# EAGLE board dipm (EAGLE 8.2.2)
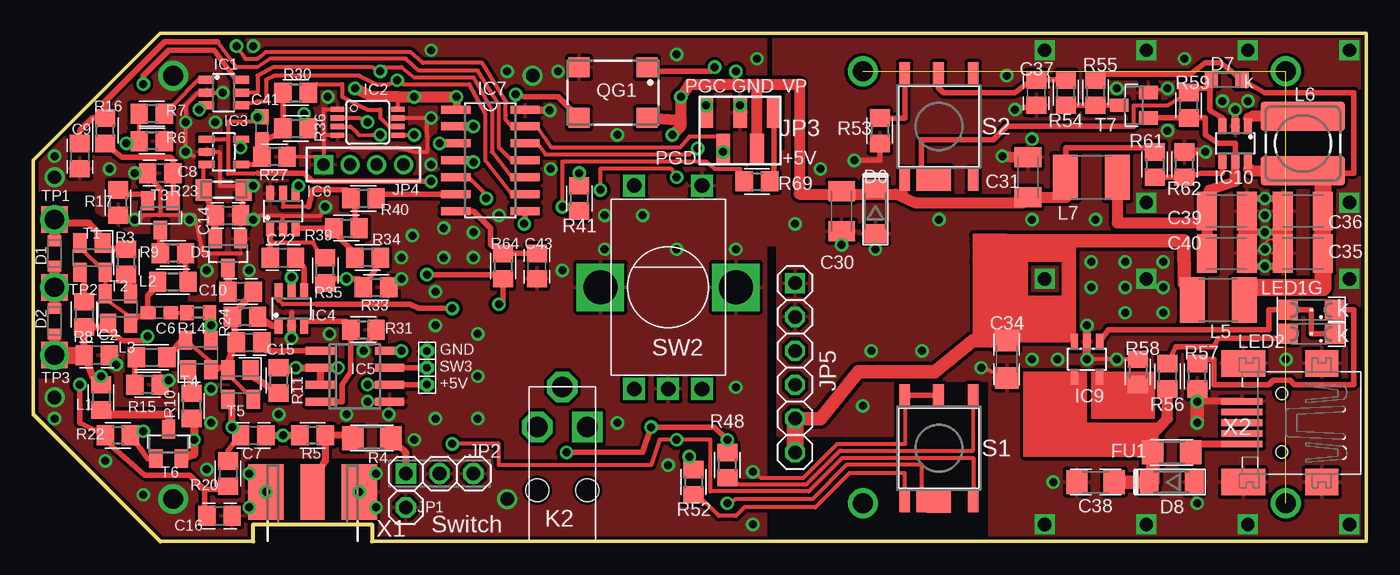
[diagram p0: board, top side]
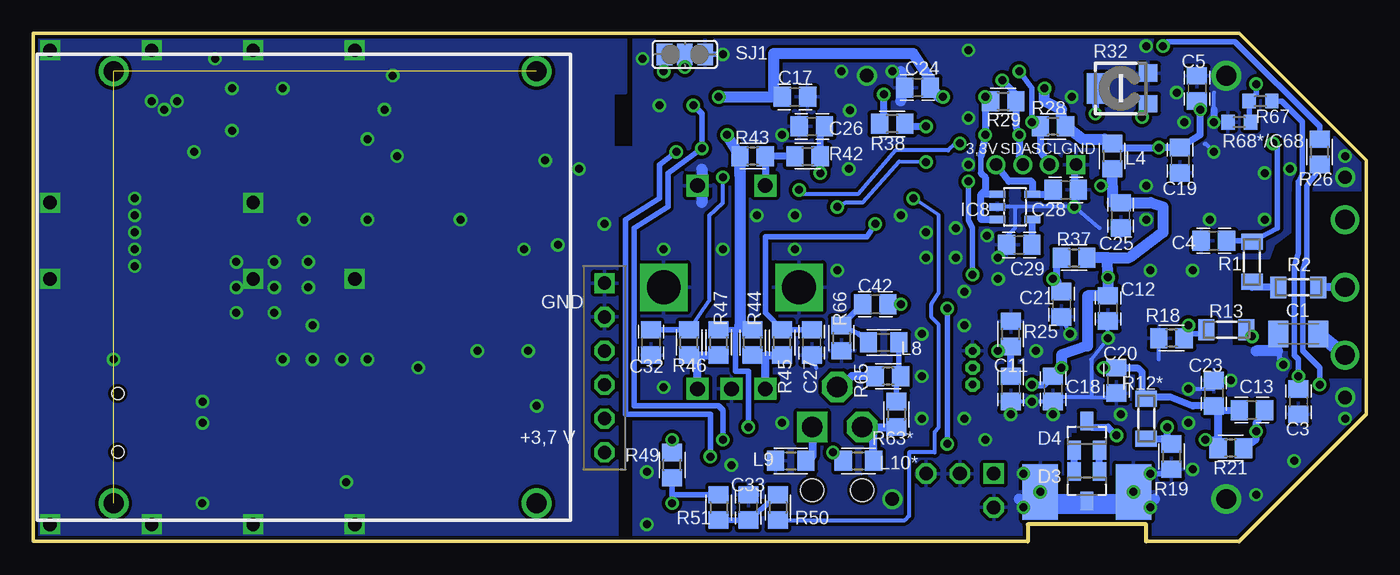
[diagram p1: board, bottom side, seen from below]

Size 100 x 38.1 mm. Coordinates in mm from the lower left corner, seen from the top.
Outline: 0,28.57 9.53,38.09 100,38.09 100,0 25.4,0 25.4,1.27 16.51,1.27 16.51,0 9.53,0 0,9.53 0,28.57
Outline: 0,28.57 9.53,38.1
Copper layers (1*16): Top 0.035mm / dielectric 1.5mm / Bottom 0.035mm
Design rules "default *": minimum track width 6mil, minimum drill 0.35mm, track to track 8mil, track to pad 8mil, pad to pad 8mil, via to via 8mil, smd to smd 0mil, copper to edge 6mil, drill to drill 6mil, minimum pad ring 10mil, minimum via ring 8mil, stop-mask expansion 4mil, vias tented up to drill 0mil, thermal gap 10mil

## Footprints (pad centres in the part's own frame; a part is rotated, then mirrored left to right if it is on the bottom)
C1206K = smd 1.5 x 2: 1 -1.5,0; 2 1.5,0
C0805 = smd 1.3 x 1.5: 1 -0.95,0; 2 0.95,0
C0603 = smd 1.1 x 1: 1 -0.85,0; 2 0.85,0
C1206 = smd 1.6 x 1.8: 1 -1.4,0; 2 1.4,0
C1210K = smd 1.5 x 2.9: 1 -1.5,0; 2 1.5,0
VARICAP = smd 0.8 x 1: A 0.95,0; C -0.95,0
SOT23 = smd 1 x 1.4: 1 -0.95,-1.1; 2 0.95,-1.1; 3 0,1.1
SOD80C = smd 1.4 x 1.8: A 1.7,0; C -1.7,0
DIODE = smd 1 x 1.2: A 1.15,0; C -1.15,0
R1206 = smd 1.6 x 1.803: 1 -1.422,0; 2 1.422,0
SOT23-6 = smd 0.6 x 1.194: 1 -0.95,-1.3; 2 0,-1.3; 3 0.95,-1.3; 4 0.95,1.3; 5 0,1.3; 6 -0.95,1.3
MSOP08 = smd 0.4 x 1: 1 -0.976,-2.263; 2 -0.326,-2.263; 3 0.324,-2.263; 4 0.974,-2.263; 5 0.974,2.262; 6 0.324,2.262; 7 -0.326,2.262; 8 -0.976,2.262
SOT232-5 = smd 0.55 x 1.2: 1 -0.95,-1.3; 2 0,-1.3; 3 0.95,-1.3; 4 0.95,1.3; 5 -0.95,1.3
SO08 = smd 0.6 x 2.2: 1 -1.905,-2.6; 2 -0.635,-2.6; 3 0.635,-2.6; 4 1.905,-2.6; 5 1.905,2.6; 6 0.635,2.6; 7 -0.635,2.6; 8 -1.905,2.6
SO14 = smd 0.6 x 2.2: 1 -3.81,-2.6; 2 -2.54,-2.6; 3 -1.27,-2.6; 4 0,-2.6; 5 1.27,-2.6; 6 2.54,-2.6; 7 3.81,-2.6; 8 3.81,2.6; 9 2.54,2.6; 10 1.27,2.6; 11 0,2.6; 12 -1.27,2.6; 13 -2.54,2.6; 14 -3.81,2.6
1X01 = drill 1.016 octagon: 1 0,0
1X03-S = drill 1.016 square: 1 -2.54,0 | drill 1.016 octagon: 2 0,0; 3 2.54,0
PIN5 = smd 1.016 x 2.2: 1 -1.905,1.33; 2 -0.635,-1.33; 3 0.635,1.33; 4 1.905,-1.33; 5 3.175,1.33
1X04M = drill 0.914 square: 1 -3,0 | drill 0.914: 2 -1,0; 3 1,0; 4 3,0
1X06-S = drill 1 square: 1 -6.35,0 | drill 1 octagon: 2 -3.81,0; 3 -1.27,0; 4 1.27,0; 5 3.81,0; 6 6.35,0
K1501-5 = drill 1.524 square: 1 -1.875,-3.5 | drill 1.524 octagon: 2 0,-6.5; 3 1.875,-3.5 | hole 1.702: -1.875,1.25; 1.875,1.25
0805 = smd 1.3 x 1.5: 1 -0.95,0; 2 0.95,0
COIL1 = smd 1.3 x 1.5: 1 -1.143,0; 2 1.143,0
L1812 = smd 1.9 x 3.4: 1 -1.95,0; 2 1.95,0
POWER-CHOKE_WE-TPC = smd 6.3 x 2.2: 1 0,2.05; 2 0,-2.05
SML1206 = smd 1.5 x 1.5: A 1.75,0; C -1.75,0
SM77H = smd 1.6 x 1.5: 1 -2.55,-1.9; 2 2.55,-1.9; 3 2.55,1.9; 4 -2.55,1.9
MINI_MELF-0204W = smd 1.2 x 1.6: 1 -1.5,0; 2 1.5,0
R0805 = smd 1.3 x 1.5: 1 -0.95,0; 2 0.95,0
R0603 = smd 1 x 1.1: 1 -0.85,0; 2 0.85,0
RTRIMCVR42A = smd 1.3 x 1.4: 1 -1.15,-2.05; 3 1.15,-2.05 | smd 2.3 x 1.5: 2 0,1.8
DTSM-6 = smd 1.676 x 0.813: 1G+ -3.975,2.567; 2G- 3.975,2.567; 3R- -3.975,-2.567; 4R+ 3.975,-2.567; 5 -3.975,1.298; 6 3.975,0.028
SJ_2 = smd 1.168 x 1.6: 1 -1.524,0; 2 0,0; 3 1.524,0
ALPS_EC12E_SW = drill 2.54 square: 1 -5.08,0; 2 5.08,0 | drill 1.1 square: A -2.54,-7.62; B 2.54,-7.62; C 0,-7.62; D -2.54,7.635; E 2.54,7.635
SOT143 = smd 1.2 x 1.44: 1 -0.75,-1.1 | smd 1 x 1.44: 2 0.95,-1.1; 3 0.95,1.1; 4 -0.95,1.1
TP20SQ = smd 2 x 2: TP 0,0
TP18SQ = smd 1.8 x 1.8: TP 0,0
PINHD1X01V = drill 0.559 pad 0.914 octagon: 1 0,0
J502-ND-142-0711-821/826 = smd 4.191 x 1.778: 1 2.115,0 | smd 4.191 x 2.667: G@1 2.115,3.495; G@2 2.115,-3.495 | smd 4.191 x 2.667 bottom: G@3 2.115,3.495; G@4 2.115,-3.495
32005-301 = smd 3.1 x 0.5: 1 3,1.6; 2 3,0.8; 3 3,0; 4 3,-0.8; 5 3,-1.6 | smd 2.5 x 2: M1 -3,-4.45; M2 -3,4.45 | smd 3.3 x 2: M3 2.9,4.45; M4 2.9,-4.45 | hole 0.9: 0,2.2; 0,-2.2

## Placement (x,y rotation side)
C1  100n  [C1206K]  5.08,15.56 0 bottom
C2  10n  [C0805]  4.76,13.97 180 top
C3  4u7  [C0805]  5.08,10.48 90 bottom
C4  100n  [C0805]  11.43,22.54 0 bottom
C5  100n  [C0805]  12.7,33.97 270 bottom
C6  2n2  [C0603]  9.47,17.14 0 top
C7  2n2  [C0805]  16.51,7.94 0 top
C8  470n  [C0805]  9.53,27.62 0 top
C9  47n  [C0805]  3.49,28.89 270 top
C10  2j2  [C0805]  15.56,18.73 0 top
C11  1n  [C0805]  26.67,11.43 90 bottom
C12  4u7  [C0805]  19.37,17.46 270 bottom
C13  100n  [C0805]  8.57,9.84 0 bottom
C14  100  [C0805]  14.61,24.45 0 top
C15  1n  [C0805]  16.19,14.92 0 top
C16  470n  [C0805]  13.97,1.9 180 top
C17  100n  [C0805]  42.86,33.34 0 bottom
C18  100n  [C0805]  23.5,11.43 270 bottom
C19  1u  [C0805]  13.97,28.57 270 bottom
C20  4u7  [C0805]  18.73,12.06 270 bottom
C21  4u7  [C0805]  22.86,17.78 90 bottom
C22  2n2  [C0805]  18.73,21.27 180 top
C23  1u  [C0805]  11.43,11.11 90 bottom
C24  1u  [C0805]  33.66,34.04 0 bottom
C25  1u  [C0805]  18.41,24.45 270 bottom
C26  22n  [C0805]  41.59,31.11 180 bottom
C27  10n  [C0805]  41.59,14.92 270 bottom
C28  4u7  [C0805]  22.54,26.35 180 bottom
C29  10n  [C0805]  26.04,22.23 180 bottom
C30  10u  [C1206K]  60.64,24.77 90 top
C31  10u  [C1206K]  74.61,27.3 270 top
C32  10n  [C0805]  53.66,14.92 270 bottom
C33  10n  [C0805]  46.35,2.54 90 bottom
C34  4u7  [C1206]  73.03,13.65 270 top
C35  10u  [C1210K]  95.25,21.59 180 top
C36  10u  [C1210K]  95.25,24.77 180 top
C37  2u2  [C0805]  75.25,33.66 270 top
C38  4u7  [C1206]  79.69,4.45 180 top
C39  10u  [C1210K]  89.53,24.77 0 top
C40  10u  [C1210K]  89.53,21.59 0 top
C41  2n2  [C0603]  17.14,30.99 90 top
C42  470n  [C0805]  36.83,17.78 180 bottom
C43  4u7  [C0805]  37.78,20.64 90 top
D1  BBY5303  [VARICAP]  1.59,21.59 270 top
D2  BBY5303  [VARICAP]  1.59,16.51 90 top
D3  BAR63-04  [SOT23]  20.95,4.13 180 bottom
D4  BAR63-04  [SOT23]  20.95,7.94 0 bottom
D5  HSMS-2822  [SOT23]  14.61,21.59 180 top
D6  5V1  [SOD80C]  63.18,24.77 270 top
D7  1N4148  [DIODE]  89.53,34.61 180 top
D8  5V6  [SOD80C]  85.41,4.45 0 top
FU1  0,3A  [R1206]  85.41,6.67 180 top
IC1  MCP4726  [SOT23-6]  14.29,33.66 270 top
IC2  MCP4551-103  [MSOP08]  25.08,31.43 270 top
IC3  MCP6271  [SOT232-5]  14.29,29.21 270 top
IC4  NC7SB3157P6  [SOT23-6]  19.37,17.46 0 top
IC5  MC12080D  [SO08]  24.13,12.38 270 top
IC6  TLV3501  [SOT23-6]  18.73,24.77 0 top
IC7  PIC16F1705  [SO14]  34.29,28.57 270 top
IC8  LP2985-3  [SOT232-5]  26.35,25.08 270 bottom
IC9  MCP73831  [SOT232-5]  79.06,13.65 180 top
IC10  MCP1640  [SOT23-6]  90.17,29.85 180 top
JP1  PINHD-1X01_2.54  [1X01]  27.94,2.54 0 top
JP2  [1X03-S]  30.48,5.08 0 top
JP3  [PIN5]  52.39,30.8 0 top
JP4  [1X04M]  24.77,28.26 0 top
JP5  [1X06-S]  57.15,13.02 270 top
K2  [K1501-5]  39.69,5.08 180 top
L1  COIL  [0805]  5.08,10.79 270 top
L2  [COIL1]  10.48,19.47 0 top
L3  [COIL1]  8.89,13.8 0 top
L4  COIL  [0805]  19.05,28.89 90 bottom
L5  1uH  [L1812]  88.9,18.1 180 top
L6  4,7uH  [POWER-CHOKE_WE-TPC]  95.25,29.85 0 top
L7  47uH  [L1812]  79.38,27.3 0 top
L8  [COIL1]  36.2,14.92 0 bottom
L9  [COIL1]  43.18,6.03 0 bottom
L10*  [COIL1]  38.1,6.03 0 bottom
LED1G  HSMF-C115  [SML1206]  95.89,17.36 180 top
LED2  [SML1206]  95.89,15.57 180 top
QG1  SM77H  [SM77H]  43.5,33.66 180 top
R1  33k  [MINI_MELF-0204W]  8.57,20.96 90 bottom
R2  M15  [MINI_MELF-0204W]  5.08,19.05 180 bottom
R3  10  [R0805]  6.99,20.96 90 top
R4  51  [R1206]  25.4,7.75 0 top
R5  47  [R0805]  20.95,7.94 180 top
R6  47k  [R0805]  8.89,30.02 180 top
R7  10k  [R0805]  8.89,32.07 180 top
R8  10  [R0805]  3.81,17.02 270 top
R9  560  [R0805]  10.48,21.59 180 top
R10  10  [R0805]  11.87,10.16 270 top
R11  10  [R0805]  18.41,12.06 270 top
R12*  [MINI_MELF-0204W]  16.51,9.21 270 bottom
R13  22k  [MINI_MELF-0204W]  10.48,15.87 180 bottom
R14  100  [R0603]  12.38,17.14 0 top
R15  560  [R0805]  8.57,11.75 180 top
R16  100k  [R0805]  5.4,30.8 90 top
R17  100  [R0805]  6.35,25.4 270 top
R18  33k  [R0805]  14.61,15.24 180 bottom
R19  33k  [R0805]  14.61,6.35 270 bottom
R20  22k  [R0805]  14.61,5.08 270 top
R21  220k  [R0805]  10.16,6.98 180 bottom
R22  12k  [R0805]  6.35,7.94 180 top
R23  5M6  [MINI_MELF-0204W]  14.29,26.35 180 top
R24  1k  [R0805]  15.88,16.83 180 top
R25  M39  [R0805]  26.67,15.56 90 bottom
R26  220  [R0805]  3.49,29.21 90 bottom
R27  1k  [R0805]  18.1,28.83 180 top
R28  10k  [R0805]  23.5,31.11 180 bottom
R29  10k  [R0805]  27.23,33.02 0 bottom
R30  27k  [R0805]  19.68,33.66 0 top
R31  820  [R0805]  24.77,15.87 0 top
R32  10k  [RTRIMCVR42A]  18.41,33.97 90 bottom
R33  8k2  [R0805]  25.72,19.05 0 top
R34  12k  [R0805]  25.08,21.27 180 top
R35  12k  [R0805]  21.91,20.32 90 top
R36  27k  [R0805]  19.68,30.98 0 top
R37  8k2  [R0805]  21.91,21.27 0 bottom
R38  100  [R0805]  35.56,31.31 180 bottom
R39  1M  [R0805]  23.5,23.5 0 top
R40  100  [R0805]  24.77,25.72 0 top
R41  6k8  [R0805]  40.96,25.72 270 top
R42  2k2  [R0805]  41.91,28.89 0 bottom
R43  5k6  [R0805]  46.04,28.89 180 bottom
R44  10k  [R0805]  46.04,14.92 90 bottom
R45  10k  [R0805]  43.81,14.92 90 bottom
R46  10k  [R0805]  50.8,14.92 90 bottom
R47  10k  [R0805]  48.58,14.92 90 bottom
R48  1k2  [R0805]  52.07,5.71 90 top
R49  10k  [R0805]  52.07,5.71 90 bottom
R50  10k  [R0805]  44.13,2.54 270 bottom
R51  10k  [R0805]  48.58,2.54 270 bottom
R52  680  [R0805]  49.53,4.45 270 top
R53  680  [R0805]  63.5,30.8 270 top
R54  M22  [R0805]  77.47,33.66 90 top
R55  M15  [R0805]  79.69,33.66 270 top
R56  1k2  [R0805]  85.09,12.38 270 top
R57  680  [R0805]  87.31,12.38 90 top
R58  6k8  [R0805]  82.87,12.7 270 top
R59  M82  [R0805]  86.68,32.7 90 top
R61  47k  [R0805]  84.14,28.26 270 top
R62  15k  [R0805]  86.36,28.26 90 top
R63*  220  [R0805]  35.24,9.53 270 bottom
R64  4k7  [R0805]  35.24,20.64 270 top
R65  220  [R0805]  35.88,12.38 180 bottom
R66  220k  [R0805]  39.37,15.24 270 bottom
R67  1k2  [R0603]  7.94,33.02 180 bottom
R68*/C68  220n  [R0603]  9.53,31.43 180 bottom
R69  100  [R0805]  54.29,26.99 0 top
S1  DTSM-6  [DTSM-6]  67.94,6.98 90 top
S2  DTSM-6  [DTSM-6]  67.94,31.11 90 top
SJ1  [SJ_2]  51.12,36.51 180 bottom
SW2  EC12E_SW  [ALPS_EC12E_SW]  47.62,19.05 0 top
T1  BFT182TW  [SOT143]  4.45,21.27 180 top
T2  BFT182TW  [SOT143]  6.35,17.46 0 top
T3  BFR93  [SOT23]  9.53,24.45 180 top
T4  BFT182TW  [SOT143]  12.38,13.97 0 top
T5  BFT182TW  [SOT143]  15.56,11.75 180 top
T6  BSS83P  [SOT23]  10.16,7.3 0 top
T7  2N7002  [SOT23]  82.55,32.7 90 top
TP1  TPSQTP20SQ  [TP20SQ]  1.59,24.13 0 top
TP2  TPSQTP20SQ  [TP20SQ]  1.59,19.05 0 top
TP3  TPSQTP20SQ  [TP20SQ]  1.59,13.97 0 top
TP4  TPTP18SQ  [TP18SQ]  67.94,27.18 0 top
TP5  TPTP18SQ  [TP18SQ]  67.94,3.05 0 top
U$1  PINHD1X1V  [PINHD1X01V]  29.53,11.75 0 top
U$3  PINHD1X1V  [PINHD1X01V]  29.53,14.29 0 top
U$4  PINHD1X1V  [PINHD1X01V]  29.53,13.02 0 top
X1  MCX/SMA  [J502-ND-142-0711-821/826]  20.95,1.59 90 top
X2  MINI-USB  [32005-301]  93.66,8.89 180 top

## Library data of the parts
C1-C43 FU1 L5-L7 R1-R11 R12* R13-R59 R61 R62 R63* R64-R67 R68*/C68 R69 = rcl
D1 D2 D7 IC1-IC4 IC6-IC10 JP3 K2 L1-L4 L8 L9 L10* T3 T6 T7 = pdk1
D3-D6 D8 = diode
IC5 = on-semiconductor; MF: ON SEMICONDUCTOR; MPN: MC12080D; OC_FARNELL: 1607924; OC_NEWARK: 40C2542
JP1 JP2 JP4 JP5 U$1 U$3 U$4 = pinhead-2
LED1G LED2 = led
QG1 = crystal; OC_FARNELL: unknown; OC_NEWARK: unknown
S1 S2 = switch-led
SJ1 = jumper
SW2 = switch-alps_1; MPN: EC12E2424407; OC_FARNELL: 1520813; OC_NEWARK: 74M1068
T1 T2 T4 T5 = transistor
TP1-TP5 = testpad
X1 = con-coax; MF: JOHNSON COMPONENTS; MPN: 142-0711-821; OC_FARNELL: 1019328; OC_NEWARK: 16F3627
X2 = con-cypressindustries; OC_FARNELL: unknown; OC_NEWARK: unknown

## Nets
DAC8: C9.1 IC7.11 R16.2
GND: C1.1 C2.1 C3.1 C4.1 C5.1 C8.1 C9.2 C11.1 C12.2 C14.2 C16.1 C17.2 C18.2 C19.2 C20.2 C21.1 C23.2 C24.1 C25.2 C26.2 C27.2 C28.1 C29.2 C30.1 C31.1 C32.2 C33.2 C34.2 C35.2 C36.2 C37.2 C38.2 C39.2 C40.2 C43.1 D3.3 D5.1 D6.A D8.A IC1.2 IC2.1 IC2.4 IC2.7 IC3.2 IC4.2 IC5.5 IC6.2 IC6.6 IC7.14 IC8.2 IC9.2 IC10.2 JP1.1 JP2.2 JP2.3 JP3.3 JP4.1 JP5.1 JP5.2 L9.1 QG1.2 R6.1 R15.1 R17.2 R18.2 R19.2 R23.1 R25.2 R27.1 R31.2 R32.3 R33.2 R53.2 R57.1 R58.1 R62.2 R66.2 R68*/C68.2 S1.2G- S1.6 SJ1.1 SW2.1 SW2.2 SW2.C SW2.E T7.2 U$3.1 X1.G@1 X1.G@2 X1.G@3 X1.G@4 X2.5 X2.M1 X2.M2 X2.M3 X2.M4
IN+: C41.2 C42.1 IC3.1 R32.1 R64.2
N$1: D1.C R3.2 T1.1 TP1.TP
N$2: C10.1 D5.3
N$3: D1.A D2.A R2.1 TP2.TP
N$4: R8.1 T1.3
N$5: C6.1 L2.1 T1.2 T1.4 T2.2 T2.4
N$6: R3.1 T2.3
N$7: C43.2 IC7.7 R64.1
N$8: IC7.6 R40.2
N$9: L2.2 R9.1
N$10: R1.1 R2.2
N$11: R13.2 R14.2 R18.1 T4.3
N$12: R10.1 T4.1
N$13: C10.2 C15.1 L3.2 R24.2 T4.2 T4.4 T5.2 T5.4
N$14: R17.1 T3.2
N$15: C15.2 IC5.1
N$16: C8.2 R16.1 T3.1
N$17: R9.2 T3.3
N$18: C11.2 IC5.8 R25.1
N$19: IC4.1 R24.1
N$20: IC4.3 IC5.4 R31.1
N$21: C22.2 IC6.1 R35.2
N$22: C22.1 IC4.4
N$23: IC6.3 R34.2 R39.1
N$24: C7.2 D4.3 R5.2
N$25: R4.1 R5.1 X1.1
N$26: IC6.5 R39.2 R40.1
N$27: C21.2 R33.1 R34.1 R35.1 R37.1
N$28: R11.2 T5.1
N$29: L3.1 R15.2
N$30: QG1.1 SJ1.2
N$31: C4.2 R1.2 R6.2 R7.2
N$32: C7.1 R12*.2 R19.1 R20.1 T5.3
N$33: L1.2 T6.3
N$34: C13.2 R21.1 R22.1 T6.1
N$35: IC5.7 U$4.1
N$36: D3.2 D4.1
N$37: D3.1 D4.2
N$38: C6.2 R14.1
N$39: IC1.6 R67.2 R68*/C68.1
N$40: JP2.1 R4.2
N$41: C16.2 R20.2 R22.2 R26.1
N$42: K2.3 L10*.2 R63*.2
N$44: C1.2 C2.2 C3.2 D2.C L1.1 R8.2 R13.1 R67.1 T2.1 TP3.TP
N$49: JP3.5 R69.2
N$57: R49.1 R51.1 S1.5 TP5.TP
N$58: IC1.1 R7.1
N$59: C14.1 D5.2 IC3.3 R23.2
N$60: IC7.4 R41.2 R69.1
N$61: C41.1 IC3.4 R27.2 R30.1 R36.1
N$62: C27.1 IC7.8 R45.2
N$63: IC7.2 R38.1
N$64: C26.1 R41.1 R42.2
N$67: C29.1 IC8.4
N$68: R42.1 R43.1 SW2.D
N$69: QG1.3 R38.2
N$70: R44.1 R45.1 SW2.A
N$71: R46.1 R47.1 SW2.B
N$72: C33.1 R50.1 R51.2
N$73: R32.2 R36.2
N$74: IC10.1 L6.1
N$75: C35.1 C36.1 D7.C IC10.6 L5.1 L6.2 R55.1
N$76: IC2.6 R30.2
N$77: D7.A IC10.3 R59.2 S2.5 TP4.TP
N$78: C39.1 C40.1 IC10.5 L7.2 R59.1 T7.1
N$79: C34.1 IC9.3 JP5.5 JP5.6 L5.2
N$80: K2.2 R65.2
N$81: IC9.5 R58.2
N$82: C37.1 R54.2 S2.6
N$83: IC10.4 R61.2 R62.1
N$84: FU1.1 X2.1
N$85: C38.1 D8.C FU1.2 IC9.4 R56.2
N$86: R54.1 R55.2 T7.3
N$87: IC9.1 LED1G.A LED2.C
N$88: LED1G.C R57.2
N$89: LED2.A R56.1
N$91: R53.1 S2.2G-
N$93: R52.2 S1.1G+
N$94: IC7.13 JP3.2 R26.2 R52.1
N$95: R48.1 S1.4R+
N$96: IC4.6 IC7.12 JP3.1 S1.3R-
N$97: C42.2 L8.1 R66.1
N$100: L8.2 R63*.1 R65.1
N$101: K2.1 L9.2
N$102: C32.1 IC7.3 R46.2
N$103: IC7.5 R50.2
SCL: IC1.5 IC2.2 IC7.10 JP4.2 R28.2
SDA: IC1.4 IC2.3 IC7.9 JP4.3 R29.2
V3.3: C28.2 IC8.5 JP4.4
VCC: C5.2 C17.1 C19.1 C24.2 C30.2 C31.2 D6.C IC1.3 IC2.5 IC2.8 IC3.5 IC7.1 IC8.1 IC8.3 JP3.4 L4.2 L7.1 L10*.1 QG1.4 R28.1 R29.1 R43.2 R44.2 R47.2 R48.2 R49.2 R61.1 S2.1G+ SJ1.3
VDD: C12.1 C13.1 C18.1 C20.1 C23.1 C25.1 IC4.5 IC5.2 IC5.3 IC5.6 IC6.4 L4.1 R10.2 R11.1 R12*.1 R21.2 R37.2 T6.2 U$1.1

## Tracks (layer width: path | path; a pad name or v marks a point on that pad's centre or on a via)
DAC8
  Top 0.305: 13.84,37.46 15.24,35.56 16.83,35.56 17.78,36.2 27.94,36.2 28.89,35.31 33.34,35.31 34.92,32.7 34.92,29.53 35.88,28.57 IC7.11
  Top 0.406: 13.84,37.46 9.84,37.46 5.4,33.02 R16.2 4.44,31.75 3.49,30.8 C9.1
GND  (via drill 0.6, 1, 1.5)
  Top 0.152: 91.03,21.04 C40.2 91.03,21.04 | 91.03,21.04 91.06,21.02 92.69,22.64 93.57,22.64 93.88,22.96 93.88,23.16 | 93.88,23.16 93.88,23.4 | 93.88,23.4 93.78,23.5 | C36.2 93.75,23.53 93.88,23.4 | 93.88,23.4 93.88,23.16 | 91.03,21.04 91.44,20.64 | C35.2 93.75,22.77 93.34,23.18 | C39.2 91.03,25.31 91.44,25.72
  Top 0.305: 10.16,29.85 R6.1 | v14.22,33.66 IC1.2 12.38,33.66 11.43,32.7 v11.43,31.43 v11.43,29.21 12.06,28.89 | v16.51,24.13 15.66,24.13 15.55,24.34 | 18.7,24.42 17.02,24.42 | 18.7,24.42 21.56,24.42 v21.91,25.08 | 18.7,23.62 18.7,24.42 | T7.2 84.14,33.82 v85.09,33.97 | R58.1 81.6,13.65 v79.06,13.65 | R57.1 v87.31,10.49 v87.31,10.48 | C34.2 v71.12,13.02 | C14.2 R23.1 v16.51,26.67 13.97,26.67 13.97,29.21 IC3.2 | 9.51,24.45 12.06,24.45 12.7,21.59 15.56,21.59 | 9.51,26.35 9.51,24.45 | v6.22,13.26 6.03,13.65 | v10.16,12.06 R15.1 | R27.1 21.77,28.89 21.77,30.46 | IC2.4 21.77,30.46 | 9.51,24.45 8.26,24.45 7.94,24.13 | IC2.7 29.52,31.75 29.53,29.21 28.64,29.21 28.18,29.32 27.36,29.53 23.81,29.53 | IC2.1 21.77,32.41 21.77,30.46 | S1.2G- 65.41,10.64 65.41,7.3 60.33,7.3 60.29,7.27 60.28,7.27 57.77,4.76 54.61,4.76 v53.98,5.21
  Top 0.406: v73.66,32.38 C37.2 | R53.2 63.5,28.57 v61.59,28.57 | D6.A v63.18,21.91 | C8.1 9.51,26.35 | v19.37,15.24 IC4.2 19.37,17.14 | R17.2 6.67,24.13 v7.62,24.13 7.94,24.13 | IC5.5 v25.08,10.48 | S1.2G- S1.6 | v24.77,14.29 25.08,14.85 25.19,14.96 25.51,15.35 R31.2
  Top 0.508: IC10.2 v90.17,32.38 | X2.5 v87.31,10.49 | C2.1 v6.22,13.26 | 91.44,20.64 93.34,20.64 | 93.34,23.18 91.44,23.18 | 91.44,25.72 93.34,25.72
  Top 0.61: v87.95,29.21 R62.2 | v79.06,13.65 IC9.2 v79.06,16.19 | IC7.14 v38.73,32.32
  Top 0.813: C30.1 v60.64,22.23 | v72.71,28.89 73.98,28.81 C31.1
  Top 1.016: v87.31,8.89 v87.31,10.49 | v87.31,10.48 R57.1
  Top 1.27: C40.2 C39.2 | 93.66,23.5 93.84,23.18 | C36.2 C35.2
  Bottom 0.305: 15.56,13.65 15.56,14.92 15.55,14.93 | 11.43,32.39 11.43,33.66 | v11.43,29.21 12.06,29.85 12.12,29.79 | 26.35,25.08 26.35,23.5 26.98,22.86 C29.2 | 26.35,25.08 IC8.2 | 20,23.5 v21.91,25.08 | v21.91,25.08 21.91,26.35 C28.1 | JP4.1 21.91,27.94 | v21.91,25.08 26.35,25.08 | C12.2 v19.37,15.24 20.64,13.65 20.64,10.79 | D3.3 20.32,2.54 | C20.2 19.37,10.8 20.64,10.79 | 20.64,10.79 23.18,10.79 C18.2 23.81,10.48 v25.08,10.48 C11.1 | v13.34,11.43 11.43,11.43 C23.2 11.11,12.06 v10.16,12.06 | v22.23,15.56 C21.1 | C27.2 41.27,13.02
  Bottom 0.406: SJ1.1 v48.26,36.51 | v16.19,5.08 14.61,5.08 R19.2 | X1.G@2 24.13,4.02 26.04,3.18 | C1.1 6.48,13.52 v6.22,13.26
  Bottom 0.508: 11.43,32.39 v11.43,31.43 | 21.91,27.94 21.91,26.35
  Bottom 0.813: 26.04,3.18 15.88,3.18 | 6.67,14.29 8.26,14.29 | 34.92,35.24 34.92,33.02 | 49.85,27.94 49.85,25.4
  Bottom 1.016: v16.19,2.54 20.32,2.54 v25.72,2.54
  other vias: 11.75,24.13 1.59,9.21 13.02,5.4 5.4,6.03 10.48,3.18 43.81,8.89 8.26,3.49 13.02,20.32 7.62,27.62 16.19,20.32 23.5,9.53 13.34,8.89 29.84,28.26 10.48,34.92 25.72,5.08 29.84,31.75 18.41,9.53 42.86,21.91 33.34,15.56 54.29,36.2 17.46,3.7 52.7,21.91 48.26,21.91 35.56,35.24 45.72,24.45 42.86,24.45 43.81,30.48 92.39,21.91 86.36,36.2 92.39,24.45 92.39,23.18 87.31,2.86 81.28,13.65 93.98,13.65 76.83,13.65 74.93,30.16 91.12,33.02 89.22,33.02 85.09,30.8 76.52,4.45 66.68,14.29 62.23,10.16 62.87,14.29 79.38,19.05 79.38,20.96 81.92,17.14 84.78,17.14 81.92,19.05 81.92,20.96 84.78,20.96 84.78,19.05 81.28,33.97 5.71,27.94 1.59,28.89 30.16,9.21 30.16,18.73 74.93,13.65 92.39,20.64 92.39,25.71 73.03,34.92 59.05,27.94 57.15,23.81 26.67,9.53 33.34,9.21 33.34,12.38 27.62,21.27 24.45,3.7 28.45,22.92 37.47,34.92 35.56,3.18 53.98,1.27 47.62,5.71 22.1,33.34 27.62,19.69 79.69,24.13 74.93,24.13 67.95,24.13 33.02,23.18 39.69,20.32 28.57,7.62 30.8,23.5 29.84,36.83 16.51,37.15 52.7,11.56 1.59,10.79 1.59,27.3 33.02,21.27 30.8,21.27 34.92,24.45 38.81,27.94 13.65,31.43 30.16,16.19 75.88,1.27 83.5,1.27 75.88,36.83 83.5,36.83 98.74,36.83 98.74,1.27 91.12,1.27 91.12,36.83 98.74,25.4 98.74,19.69 83.5,19.69 83.5,25.4 53.02,32.7 39.37,35.24 75.88,19.69
  pour Top (isolate 0.254): 55.56,38.1 100.01,38.1 100.01,0 71.75,0 71.75,12.06 64.45,12.06 64.45,7.94 55.88,7.94 55.88,22.23 54.93,22.23 54.93,28.26 55.88,28.26 55.88,29.21 56.52,29.21 56.52,33.66 55.56,33.66
  pour Top (isolate 0.254): 9.53,0 16.19,0 16.19,6.35 25.72,6.35 25.72,0 54.93,0 54.93,38.1 9.53,38.1 0,28.57 0,26.35 4.76,26.35 4.76,24.77 7.3,23.18 9.53,23.18 9.53,22.23 11.75,22.23 11.75,18.1 14.29,18.1 14.29,13.97 4.45,13.97 4.45,12.06 0,12.06 0,9.53
  pour Top: 78.74,16.51 85.41,16.51 85.41,21.59 78.74,21.59
  pour Bottom (isolate 0.254): 56.2,0 100.01,0 100.01,38.1 55.56,38.1 55.56,33.66 56.52,33.66 56.52,29.53 54.93,29.53 54.93,24.45 56.2,24.45
  pour Bottom (isolate 0.254): 25.4,0 54.93,0 54.93,38.1 9.53,38.1 0,28.57 0,26.35 5.71,26.35 5.71,23.18 6.99,22.23 7.3,21.27 10.16,21.27 10.16,14.6 4.45,14.6 4.45,12.06 0,12.06 0,9.53 9.53,0 16.51,0 16.51,1.9 18.41,1.9 18.41,5.08 20.64,5.08 20.64,8.25 22.23,8.25 22.23,5.08 23.5,5.08 23.5,1.9 25.4,1.9
IN+  (via drill 0.6)
  Top 0.305: IC3.1 14.29,30.16 14.61,30.16 | 14.61,30.16 14.61,27.56 16.51,27.56 16.83,27.62 | 14.61,30.16 14.61,31.5 16.51,31.5 v16.83,31.81 16.98,31.81 C41.2
  Top 0.406: v29.84,26.99 20.95,26.99 20.32,27.62 16.83,27.62 | v29.53,20 34.93,20.01 R64.2 35.24,18.1 v34.92,17.78
  Bottom 0.305: R32.1 16.19,32.7 16.51,32.5
  Bottom 0.406: v29.53,20 29.53,23.5 29.84,24.13 v29.84,26.99 | C42.1 v34.92,17.78
  Bottom 0.508: 16.51,32.5 v16.83,31.81
N$1  (via drill 1.45)
  Top 0.305: 1.58,23.81 TP1.TP
  Top 0.508: TP1.TP 1.8,24.13 1.85,23.87 4.17,23.87 4.88,23.16 T1.1 5.66,21.91 R3.2
  Top 0.813: D1.C 1.59,23.81 1.58,23.81
  other vias: 1.59,24.13
N$2
  Top 0.508: D5.3 C10.1
N$3  (via drill 1.45)
  Top 0.305: 1.27,19.05 TP2.TP | TP2.TP 1.59,18.1 | 1.59,19.69 TP2.TP
  Top 0.813: D2.A TP2.TP | TP2.TP D1.A
  Bottom 0.61: TP2.TP R2.1
  other vias: 1.59,19.05
N$4
  Top 0.305: 3.81,19.86 T1.3
  Top 0.406: R8.1 3.81,19.86
N$5
  Top 0.305: T1.2 3.5,22.07 T1.4 5.39,20.15 T2.4 5.55,18.1 7.3,16.83 7.3,16.68 T2.2 | 7.3,16.83 T2.2 | 8.99,17.35 C6.1 8.57,17.14 | T2.2 7.52,16.68 | 9.53,19.37 L2.1
  Top 0.406: 7.52,16.68 C6.1 | 8.57,17.14 8.57,18.42 9.53,19.37
N$6
  Top 0.305: T2.3 7.3,19.79 7.2,19.79 R3.1
N$7
  Top 0.406: C43.2 R64.1 34.29,22.23 34.29,23.5 33.02,24.77 IC7.7
N$8
  Top 0.305: R40.2 26.35,26.04
  Top 0.406: 26.35,26.04 IC7.6
N$9
  Top 0.406: R9.1 11.43,20 L2.2
N$10
  Bottom 0.305: 8.57,19.05 R1.1
  Bottom 0.508: R2.2 8.57,19.05
N$11  (via drill 0.6)
  Top 0.305: R14.2 13.33,17.36 | v13.34,16.19 v13.33,16.19
  Top 0.406: 13.33,17.36 v13.33,16.19 T4.3
  Bottom 0.305: R13.2 11.74,15.56 | 13.02,15.56 13.34,15.24 R18.1 13.34,15.56 v13.34,16.19
  Bottom 0.406: 11.74,15.56 13.02,15.56
N$12
  Top 0.305: T4.1 11.5,12.55
  Top 0.508: 11.5,12.55 11.75,12.06 11.75,11.11 R10.1
N$13
  Top 0.305: 13.33,13.02 T4.2 | T4.2 13.33,12.85 | C15.1 15.09,14.78 | C15.1 15.24,14.6 | C15.1 | T4.2 14.52,12.91 13.57,13.25 T4.4 | 11.19,15.56 11.59,15 11.75,14.92 11.75,15.39 T4.4 | 14.59,13.19 T5.2 14.61,12.55 T5.4 | 11.43,15.39 T4.4
  Top 0.508: 14.52,12.91 15.09,14.78 | C15.1 R24.2 C10.2 | T4.2 14.59,13.19 | L3.2 11.43,15.39
N$14
  Top 0.305: R17.1 6.99,26.03 | 8.57,26.04 8.72,25.4 T3.2
  Top 0.406: 6.99,26.03 8.57,26.04
N$15
  Top 0.305: 17.46,14.29 C15.2
  Top 0.406: IC5.1 17.46,14.29
N$16
  Top 0.305: R16.1 5.73,29.53
  Top 0.406: 10.48,26.03 C8.2 10.47,28.58 10.25,28.8 6.68,28.8 5.73,29.53
  Top 0.508: T3.1 10.48,26.03
N$17
  Top 0.508: T3.3 9.53,22.55 R9.2
N$18  (via drill 0.6)
  Top 0.305: IC5.8 v27.62,14.29
  Bottom 0.305: R25.1 v27.62,14.29
  Bottom 0.508: C11.2 R25.1
N$19
  Top 0.508: R24.1 17.9,16.19 IC4.1
N$20
  Top 0.305: 23.81,16.19 R31.1 23.69,16.19 | 23.69,16.19 R31.1 | IC4.3 20.5,16.31 20.6,16.51 | 23.47,16.51 23.69,16.19
  Top 0.406: IC5.4 23.18,10.48 23.18,11.75 23.81,12.7 23.81,16.19 | 20.6,16.51 23.47,16.51
N$21
  Top 0.305: R35.2 21.27,21.91 21.01,22.43 17.78,22.43 17.78,22.54 | 17.78,21.59 C22.2
  Top 0.406: 17.78,21.59 17.78,22.54 | 17.78,22.43 IC6.1
N$22
  Top 0.305: C22.1
  Top 0.406: IC4.4 20.32,20.52 C22.1
N$23
  Top 0.305: R39.1 22.86,22.86 | 24.13,21.59 R34.2
  Top 0.406: 22.86,22.86 24.13,21.59 | R39.1 20.32,23.5 IC6.3
N$24  (via drill 0.6)
  Top 0.508: C7.2 v18.73,7.94 R5.2
  Bottom 0.508: D4.3 20.95,8.89 20.64,8.57 19.37,8.57 v18.73,7.94
N$25
  Top 0.305: X1.1 20.96,4.79 20.95,4.47 | R5.1
  Top 0.508: R4.1 23.5,7.94 R5.1 | R5.1 21.91,6.03 20.95,4.47
N$26
  Top 0.305: IC6.5 18.73,25.08 20.64,25.08 | R40.1 23.5,26.35
  Top 0.406: 23.5,26.35 20.95,26.35 20.64,25.08 | R39.2 24.13,24.13 24.13,25.08 R40.1
N$27  (via drill 0.6)
  Top 0.305: 25.98,20.9 26.3,20.9 26.35,20.95 R34.1
  Top 0.406: R35.1 22.23,19.69 v23.5,19.69 24.45,19.69 R33.1 25.98,20.9
  Bottom 0.305: R37.1 23.23,21.27
  Bottom 0.508: 23.23,19.7 v23.5,19.69 | 23.23,19.7 C21.2 | 23.23,21.27 23.23,19.7
N$28
  Top 0.305: R11.2 18.41,10.8 | T5.1 16.68,12.21
  Top 0.508: 16.68,12.21 R11.2
N$29
  Top 0.305: L3.1 7.62,13.65
  Top 0.406: 7.62,13.65 R15.2
N$30  (via drill 0.6)
  Top 0.305: 46.67,35.24 QG1.1
  Top 0.406: v51.12,35.56 50.8,35.24 46.67,35.24
  Bottom 0.406: SJ1.2 v51.12,35.56
N$31  (via drill 0.6)
  Top 0.305: v6.99,29.85 7.94,30.16 | 7.94,30.16 R7.2 | 8.26,30.16 7.94,30.16
  Top 0.406: R6.2 v6.99,29.85
  Bottom 0.406: v6.99,29.85 6.67,29.53 6.67,23.5 R1.2 8.66,22.54 C4.2
N$32  (via drill 0.6)
  Top 0.305: T5.3 14.61,10.48 | 15.24,8.25 C7.1 15.49,8.01
  Top 0.406: R20.1 14.61,6.81 15.49,8.01
  Top 0.508: 14.61,10.48 14.92,9.84 v14.92,8.57 15.24,8.25
  Bottom 0.508: 14.92,7.71 v14.92,8.57 | R12*.2 14.92,7.71 | 14.92,7.71 R19.1
N$33
  Top 0.508: 5.4,9.84 L1.2
  Top 0.61: L1.2 5.4,9.53 10.16,9.53 T6.3
N$34  (via drill 0.6)
  Top 0.305: R22.1 6.99,8.25 6.98,8.26 7.62,8.26 v8.26,8.25
  Top 0.406: T6.1 8.57,6.2 R22.1
  Bottom 0.508: C13.2 8.26,8.89 v8.26,8.25 8.26,7.62 R21.1
N$35
  Top 0.406: IC5.7 U$4.1
N$36
  Bottom 0.508: D3.2 D4.1
N$37
  Bottom 0.508: D3.1 D4.2
N$38
  Top 0.305: C6.2 R14.1
N$39  (via drill 0.6)
  Top 0.406: IC1.6 15.24,34.6 15.25,34.6 15.12,34.74 13.56,36.83 10.16,36.83 8.26,34.92 v8.26,34.29
  Bottom 0.406: R68*/C68.1 8.79,31.54 R67.2 8.26,33.55 v8.26,34.29
N$40
  Top 0.508: R4.2 27.94,6.67 JP2.1
N$41  (via drill 0.6)
  Top 0.305: 5.34,7.99 5.02,8 R22.2 | 14.61,3.9 R20.2
  Top 0.406: R22.2 3.49,8.89 v3.49,11.75 | 5.34,7.99 5.87,7.15 8.36,4.97 11.72,4.97 12.8,3.9 12.85,3.9 | 12.85,3.9 14.61,3.9 | C16.2 12.85,2.37 12.85,3.9
  Bottom 0.406: v3.49,11.75 3.49,13.02 4.76,14.29 4.76,20.32 4.45,21.27 4.45,26.67 3.49,27.94 R26.1
N$42
  Bottom 0.406: 36.96,8.56 37.13,8.57
  Bottom 0.61: R63*.2 37.13,8.57 37.19,8.57 K2.3 | L10*.2 36.96,8.56
N$44  (via drill 0.6, 1.45)
  Top 0.305: 1.9,14.6 TP3.TP | v5.08,12.38 5.39,11.75 L1.1 | 5.4,16.25 T2.1
  Top 0.406: 5.31,16.07 6.72,15.06 8.26,15.06 v8.57,15.37
  Top 0.508: v5.08,12.38 4.45,12.38 C2.2 3.81,15.75 R8.2 5.31,16.07 T2.1
  Top 0.813: TP3.TP D2.C
  Top 1.27: TP3.TP C2.2
  Bottom 0.305: R13.1 v8.57,15.37
  Bottom 0.406: v5.08,12.38 5.08,13.65 5.4,13.97 5.4,20.64 5.08,21.59 5.08,26.97 4.8,27.56 4.8,31.47 6.35,33.02 R67.1
  Bottom 0.508: C3.2 v5.08,12.38
  Bottom 1.016: C1.2 TP3.TP
  other vias: 1.59,13.97
N$45  (via drill 1.5)  (2 unrouted)
  other vias: 62.23,35.24 93.98,35.24 93.98,2.86
N$46  (via drill 1.5)
  other vias: 62.23,2.86
N$49
  Top 0.406: JP3.5 55.56,26.67 R69.2
N$57  (via drill 0.6)
  Top 0.305: v52.07,2.86 52.7,3.18 58.45,3.18 61.01,5.74 66.65,5.74 S1.5 67.91,3.01 TP5.TP
  Bottom 0.406: 52.07,3.49 R49.1 | 52.07,3.49 v52.07,2.86 | 52.07,3.49 51.12,3.49 50.8,3.49 R51.1
N$58
  Top 0.305: IC1.1 12.38,34.6 10.48,32.7 R7.1
N$59
  Top 0.305: D5.2 13.65,23.01 | 13.65,24.13 C14.1 | R23.2 12.79,28.14 IC3.3
  Top 0.508: 13.65,23.01 13.65,24.13 | C14.1 R23.2
N$60  (via drill 0.6)
  Top 0.305: 31.49,28.57 IC7.4 | R41.2 v39.69,25.08 39.69,28.5 50.48,28.5 51.12,27.94 53.02,27.94 53.02,26.67 R69.1
  Top 0.406: IC7.4 v33.02,28.45
  Bottom 0.305: v33.02,28.45 35.04,28.47 37.78,25.4 39.05,25.4 v39.69,25.08
N$61
  Top 0.305: 17.18,28.29 R27.2 17.46,29.21 | R36.1 18.59,30.66 | C41.1 17.25,29.95 17.46,30.16
  Top 0.406: IC3.4 17.18,28.29 | R30.1 18.73,31.43 R36.1 | 18.59,30.66 17.46,30.16 17.46,29.21
N$62  (via drill 0.6)
  Top 0.305: 36.89,24.67 IC7.8 | 36.89,23.87 v36.83,23.81
  Top 0.406: IC7.8 36.89,23.87
  Bottom 0.406: C27.1 R45.2 45.09,17.14 45.09,22.86 37.47,22.86 v36.83,23.81
N$63  (via drill 0.6)
  Top 0.305: IC7.2 31.75,31.11
  Top 0.406: IC7.2 v33.02,31.11
  Bottom 0.508: R38.1 34.29,31.11 v33.02,31.11
N$64  (via drill 0.6)
  Top 0.305: R41.1 v40.96,27.62
  Bottom 0.305: R42.2
  Bottom 0.508: R42.2 40.96,30.8 C26.1 | v40.96,27.62 R42.2
N$67
  Bottom 0.508: C29.1 25.05,23.53 IC8.4
N$68
  Bottom 0.305: SW2.D
  Bottom 0.508: R42.1 R43.1 SW2.D
N$69  (via drill 0.6)
  Top 0.406: QG1.3 39.36,33.35 36.83,33.34 v36.2,33.53
  Bottom 0.508: R38.2 36.32,31.31 36.2,31.43 v36.2,33.53
N$70
  Bottom 0.406: 45.02,13.97 R44.1
  Bottom 0.61: SW2.A 45.09,13.65 45.02,13.97 R45.1
N$71
  Bottom 0.305: R47.1 48.9,13.95 | R46.1 51.12,13.95
  Bottom 0.61: SW2.B 50.16,13.97 | 50.16,13.97 R46.1 | 50.16,13.97 R47.1
N$72
  Bottom 0.406: R51.2 C33.1 R50.1
N$73  (via drill 0.6)
  Top 0.305: R36.2 20.32,30.97 v20.32,32.07
  Bottom 0.305: R32.2 20.32,33.66
  Bottom 0.508: 20.32,33.66 v20.32,32.07
N$74
  Top 0.406: IC10.1 91.12,31.75 91.19,31.75
  Top 0.813: L6.1 91.5,31.89 91.19,31.75
N$75
  Top 0.305: 97.75,27.62 96.75,27.89 | 79.96,35.04 R55.1
  Top 0.406: 97.75,27.62 99.06,27.62 99.06,33.66 92.39,33.66 D7.C 89.1,35.88 87.95,35.88 86.82,35.04 79.96,35.04 | IC10.6 91.12,27.8 91.5,27.8
  Top 0.813: L6.2 91.5,27.8 91.19,27.94
  Top 1.016: L5.1 90.85,19.05 90.81,19.05
  Top 1.27: 90.81,19.05 96.75,19.05 C35.1 C36.1 96.75,27.89 L6.2 95.25,27.64
N$76
  Top 0.305: R30.2 21.27,34.29 23.18,34.29 23.18,33.34 25.08,32.38 26.04,32.38 26.04,31.75 26.67,31.11 IC2.6
N$77
  Top 0.305: 82.55,31.11 82.55,32.7 85.11,32.7 R59.2 | R59.2 | R59.2 | TP4.TP 66.69,27.18 S2.5
  Top 0.406: 82.55,31.11 73.03,31.11 72.05,30.14 66.65,30.14 S2.5 | R59.2 86.68,33.97 88.27,33.97 D7.A 88.27,33.66 88.27,32.38 88.39,32.27 89.22,31.75 IC10.3
N$78
  Top 0.305: R59.1 86.74,31.37 86.36,31.75
  Top 0.406: IC10.5 90.17,29.85 88.9,29.85 87.95,30.48 87.95,31.75 R59.1 | T7.1 86.36,31.75
  Top 0.508: 90.17,27.62 IC10.5
  Top 0.813: 90.17,27.62 90.17,26.99 88.27,26.35 88.03,25.8 C39.1 88.03,23.88 | 88.03,23.88 C40.1 | L7.2 81.33,23.88 88.03,23.88
N$79
  Top 0.254: 78.11,22.54 | 78.11,14.6 78.11,14.89 78.11,22.69 78.11,22.86
  Top 0.305: L5.2 86.68,18.1 86.68,19.37 | IC9.3 78.11,14.89 | 78.11,22.54 78.11,22.69
  Top 1.016: JP5.5 59.05,9.21 61.91,12.7 67.63,12.7 70.48,15.05 C34.1 73.03,22.54 78.11,22.54 86.31,22.54 86.36,19.37 86.36,19.69 L5.2
  Top 1.27: JP5.5 JP5.6
N$80
  Bottom 0.61: R65.2 38.59,12.38 K2.2
N$81
  Top 0.305: R58.2 80.01,11.75 IC9.5
N$82
  Top 0.305: 74.93,34.63 C37.1
  Top 0.406: C37.1 R54.2 | S2.6 67.92,34 68.26,33.66 73.63,33.66 74.93,34.63
N$83
  Top 0.305: 89.22,28.59 IC10.4 89.2,28.57
  Top 0.406: R61.2 R62.1 87.63,27.62 89.22,27.62 89.2,28.57
N$84
  Top 0.305: 87.32,7.29 FU1.1
  Top 0.508: X2.1 87.32,7.29
N$85
  Top 0.305: IC9.4 78.11,8.22 83.82,8.25 83.82,8.02 83.91,7.93
  Top 0.813: 83.91,7.93 85.09,9.21 R56.2
  Top 1.016: C38.1 D8.C 83.99,4.45 FU1.2 83.91,6.67 83.91,7.93
N$86
  Top 0.305: T7.3
  Top 0.406: R54.1 R55.2 T7.3
N$87
  Top 0.406: IC9.1 80.64,15.87 92.71,15.87 92.71,17.36 LED1G.A 95.89,17.36 95.89,15.57 LED2.C
N$88
  Top 0.305: 87.31,13.65 R57.2
  Top 0.406: LED1G.C 99.06,17.36 99.06,11.75 94.61,11.75 94.3,12.09 93.03,12.09 92.71,11.75 88.58,11.75 88.58,13.65 87.31,13.65
N$89
  Top 0.406: R56.1 85.72,14.6 88.58,14.6 88.9,15.24 94.14,15.24 LED2.A
N$91
  Top 0.406: R53.1 65.38,31.75 S2.2G-
N$93
  Top 0.305: S1.1G+ 65.38,5.14 61.28,5.14 58.67,2.54 53.34,2.54 52.7,1.9 51.44,1.9 49.85,3.49 R52.2
N$94  (via drill 0.6)
  Top 0.305: v15.24,37.15 15.88,36.2 16.83,36.2 17.46,36.7 28.26,36.7 29.21,35.88 33.66,35.88 35.43,33.02 35.43,31.63 | v51.75,29.21 51.75,30.35 49.21,30.35 48.51,29.53 38.89,29.53 37.78,31.11 37.09,31.11 | 35.43,31.63 35.43,31.94 | IC7.13 35.88,31.11 35.43,31.63
  Top 0.406: v49.21,6.35 R52.1 | 37.09,31.11 IC7.13 | JP3.2 51.81,29.47 v51.75,29.21
  Bottom 0.406: v15.24,37.15 14.92,37.46 9.84,37.46 3.49,31.11 R26.2 | v49.21,6.35 49.21,9.53 55.56,9.53 55.56,24.13 53.02,25.72 53.02,28.26 v51.75,29.21
N$95
  Top 0.305: S1.4R+ 70.51,6.79 60.53,6.79 60.5,6.76 60.49,6.76 57.98,4.25 53.02,4.25 R48.1
N$96  (via drill 0.6)
  Top 0.305: S1.3R- 70.51,6.25 60.7,6.25 58.19,3.75 50.8,3.75 50.8,7.62 v48.26,7.62 46.99,7.62 46.35,5.71 34.92,5.71 34.92,7.3 v31.43,7.3 | IC4.6 18.41,18.61 | 21.27,17.78 18.73,17.78 18.42,18.1 | 37.78,29.85 38.42,29.02 49.21,29.02 v49.85,29.46
  Top 0.406: 18.42,18.1 IC4.6 | 21.27,17.78 28.26,17.78 28.89,17.46 v31.43,17.46 | IC7.12 37.78,29.85 | v50.48,32.7 50.42,32.07 JP3.1
  Bottom 0.406: v31.43,7.3 v31.43,17.46 | v48.26,7.62 48.26,9.84 48.58,10.16 54.93,10.16 54.93,23.5 52.39,25.08 52.39,27.62 v49.85,29.46 49.85,32.07 v50.48,32.7
N$97
  Bottom 0.406: L8.1 38.1,15.56 R66.1 C42.2
N$100
  Bottom 0.406: L8.2 35.05,13.02 R65.1 35.24,12.38 R63*.1
N$101
  Bottom 0.406: 41.56,6.35 L9.2
  Bottom 0.61: K2.1 41.56,6.35
N$102  (via drill 0.6)
  Top 0.305: v48.26,27.3 47.87,27.94 42.52,27.94 42.52,26.33 v42.55,26.35 | IC7.3 v30.48,29.85
  Bottom 0.305: v48.26,27.3 48.26,25.38 49.3,24.43 49.3,18.08 R46.2 | v30.48,29.85 30.82,29.85 31.38,29.32 35.32,29.32 38.14,26.04 42.23,26.04 v42.55,26.35
  Bottom 0.406: R46.2 C32.1
N$103  (via drill 0.6)
  Top 0.305: v33.97,25.72 33.78,25.91 33.78,26.17 32.64,27.3 IC7.5
  Bottom 0.305: R50.2 34.61,1.59 34.29,1.9 34.29,6.67 32.38,6.67 32.38,8.2 32.11,8.52 32.11,16.29 32.61,16.79 32.61,17.82 32.07,18.68 32.07,24.45 v33.97,25.72
SCL  (via drill 0.6)
  Top 0.305: IC1.5 16.83,33.66 16.83,34.92 18.01,35.56 25.4,35.56 v26.04,35.24 26.35,35.56 27.62,35.56 28.57,34.8 33.02,34.8 34.42,32.38 34.42,29.21 35.88,27.3 IC7.10 | IC2.2 24.45,31.75 v25.07,31.44
  Bottom 0.305: 24.45,31.12 v25.07,31.44 24.44,31.43 R28.2
  Bottom 0.406: v25.07,31.44 25.08,32.07 25.08,33.97 v26.04,35.24
  Bottom 0.508: JP4.2 24.45,29.26 24.45,31.12
SDA  (via drill 0.6)
  Top 0.305: IC1.4 16.83,33.02 17.46,33.02 17.46,34.61 18.1,34.92 24.45,34.92 25.72,34.29 26.69,34.29 v27.3,34.58 27.3,34.61 27.76,34.29 32.7,34.29 33.91,32.07 33.91,28.57 35.88,26.04 IC7.9 | IC2.3 23.81,31.11 24.13,30.8 24.44,30.47 25.4,30.48 v26.04,30.48
  Bottom 0.406: v27.3,34.58 26.36,33.63 R29.2
  Bottom 0.508: R29.2 26.28,31.11 v26.04,30.48 26.04,28.85 JP4.3
V3.3
  Bottom 0.305: 25.05,26.96 25.08,26.99 | 23.81,26.03 C28.2
  Bottom 0.508: 25.05,26.96 IC8.5 23.81,26.03 | 25.08,26.99 26.81,26.99 JP4.4
VCC  (via drill 0.6)
  Top 0.254: C30.2 60.01,26.04
  Top 0.305: IC3.5 15.55,30.16 v15.56,29.53 | IC2.8 27.39,33.36 27.39,33.34 | IC2.5 27.94,30.46 v28.57,30.48 | IC7.1 31.46,32.38 31.75,32.41 | IC1.3 12.99,32.67 v12.45,32.38 | D6.C 63.13,26.46 64.72,26.04
  Top 0.406: 77.47,27.94 77.47,29.53 83.5,29.53 R61.1 | 65.38,27.1 S2.1G+ 65.38,25.72 66.12,25.4 | R48.2 v52.07,7.62 51.12,8.57 v46.35,8.57 45.72,6.67 v40.01,6.67 | 52.7,34.29 v52.7,35.24
  Top 0.61: v31.75,33.34 31.75,32.41
  Top 0.813: v24.13,33.97 25.4,33.34 27.39,33.34 v28.57,33.34 v31.75,33.34 | 54.29,34.29 52.7,34.29 49.21,34.29 v48.58,33.34 48.58,31.91 | L7.1 77.47,27.94 77.47,25.8 C31.2 74.3,25.4 66.12,25.4 64.72,26.04 60.01,26.04 57.47,26.04 57.47,34.29 54.29,34.29 | JP3.4 54.29,34.29 | 48.58,31.91 48.58,31.11 v47.94,30.48 | QG1.4 48.29,31.62 48.58,31.91
  Bottom 0.305: 19.62,30.16 L4.2 | 44.45,33.34 C17.1 | IC8.1 | R29.1 v28.57,33.34 | R44.2 46.35,15.56 46.99,16.19 47.31,15.87 | R48.2 v52.07,7.62
  Bottom 0.406: 28.89,28.89 28.89,27.62 | R47.2 47.31,15.87 | 47.31,15.87 R44.2 | L10*.1 39.05,6.35 v40.01,6.67 | 47.31,15.87 47.31,12.76 46.35,12.76 v46.35,8.57 | SJ1.3 52.64,35.31 v52.7,35.24
  Bottom 0.508: L4.2 18.73,29.53 v15.56,29.53 C19.1 12.45,30.48 v12.45,32.38 C5.2 | IC8.3 28.89,24.13 28.89,26.04 | IC8.1 28.89,26.04 | v28.57,33.34 v28.57,30.48 28.89,28.89 | 28.89,27.62 28.57,27.3 28.57,26.35 28.89,26.04
  Bottom 0.813: 44.45,33.34 44.45,36.58 33.97,36.58 32.7,34.67 C24.2 32.01,33.34 v31.75,33.34 | 46.99,27.46 46.99,16.19 | R43.2 | R43.2 46.99,27.46 | v24.13,33.97 24.13,33.02 22.86,32.38 22.86,31.75 R28.1 21.27,30.16 19.62,30.16 | v48.58,33.34 C17.1 | v47.94,30.48 R43.2 | R43.2 46.99,27.46
VDD  (via drill 0.6)
  Top 0.305: R11.1 18.73,12.7 | IC6.4 19.68,26.23 v19.89,26.67
  Top 0.406: IC5.6 U$1.1
  Top 0.508: IC5.2 v19.68,13.02 18.73,12.7 | R10.2 12.06,9.21 | IC4.5 v19.37,19.8 | IC5.2 IC5.3 | IC5.2 v22.86,13.02 | v25.08,11.75 IC5.6
  Top 0.61: 12.06,9.21 v12.06,7.62 12.06,6.52 T6.2
  Bottom 0.305: R12*.1 16.82,11.11 | 16.51,10.48 R12*.1 | 16.51,11.11 R12*.1 | 11.15,9.84 11.43,9.84 | 19.05,25.4 C25.1 | 19.05,26.67 19.05,26.68
  Bottom 0.406: 11.11,7.62 11.11,7.61
  Bottom 0.508: v19.68,13.02 C20.1 17.14,13.01 16.83,12.7 16.82,11.11 | 16.19,10.92 16.51,10.48 | 11.43,9.84 C23.1 12.93,10.16 12.94,10.17 13.03,10.17 14.61,10.79 16.42,10.79 R12*.1 | 11.15,9.84 C13.1 | v25.08,11.75 24.13,11.74 C18.1 | v19.89,26.67 19.05,26.67 | v12.06,7.62 11.11,7.62
  Bottom 0.61: R21.2 11.11,7.61 11.11,10.16 C23.1
  Bottom 0.813: L4.1 19.05,26.68 19.05,25.4 | C25.1 16.18,25.4 15.24,25.08 15.24,23.18 17.78,21.27 19.4,21.27 | 19.4,21.27 R37.2 | 19.4,21.27 v19.37,19.8 C12.1 20.91,18.41 20.91,14.66 22.86,13.98 v22.86,13.02 C18.1
(copper drawn outside any net)
  shapes: Top area x9

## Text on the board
tNames: k | PGC | GND | VP | PGD | +5V | k | k | GND | SW3 | +5V | Switch
bNames: GND | SCL | SDA | 3,3V | GND | +3,7 V
bDocu: JP5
